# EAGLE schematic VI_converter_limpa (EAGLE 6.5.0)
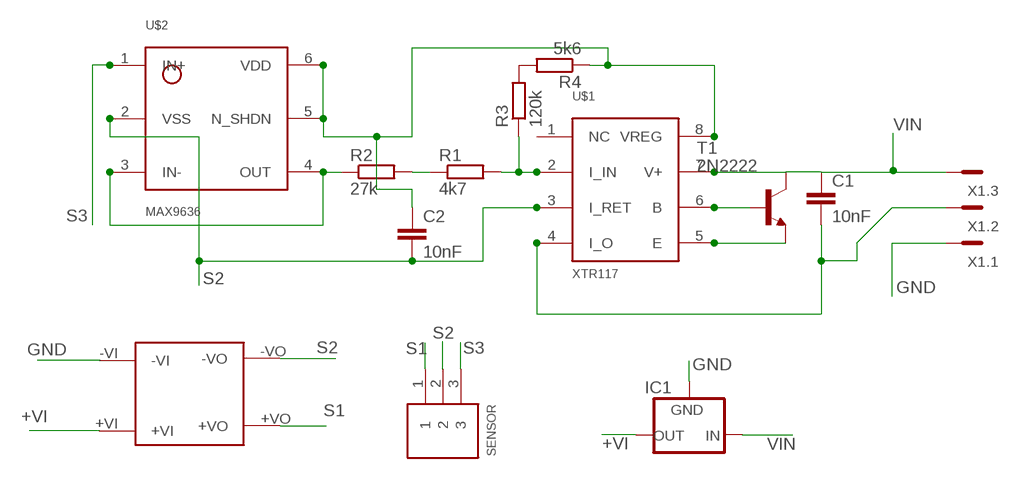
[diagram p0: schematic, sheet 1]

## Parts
C1  10nF  C-EUC1206  [C1206]
C2  10nF  C-EUC1206  [C1206]
IC1  78XXS  [78XXS]
R1  4k7  R-EU_M1206  [M1206]
R2  27k  R-EU_M1206  [M1206]
R3  120k  R-EU_M1206  [M1206]
R4  5k6  R-EU_M1206  [M1206]
SENSOR  3PIN  [B3B-PH-K-S]
T1  2N2222  [TO18]
U$1  XTR117  [MSOP8]
U$2  MAX9636  [SOT363]
U$3  ROE-0505S  [ROE-0505S]
X1  MC3  [MC3]

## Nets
GND: C2.2 U$1.3(I_RET) U$2.2(VSS) X1.1
N$1: T1.2(B) U$1.6(B)
N$2: T1.1(E) U$1.5(E)
N$4: R1.2 R3.1 U$1.2(I_IN)
N$5: R1.1 R2.2
N$6: R3.2 R4.2
N$7: C1.2 U$1.4(I_O) X1.2
N$8: R2.1 U$2.3(IN-) U$2.4(OUT)
N$14: C1.1 T1.3(C) U$1.7(V+) X1.3
S3: U$2.1(IN+)
VDD: C2.1 R4.1 U$1.8(VREG) U$2.5(N_SHDN) U$2.6(VDD)
VIN: IC1.IN
Unconnected: IC1.GND IC1.OUT SENSOR.1 SENSOR.2 SENSOR.3 U$1.1(NC) U$3.+VI U$3.+VO U$3.-VI U$3.-VO

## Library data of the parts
C1 C2 = resistor:C-EU: CAPACITOR, European symbol
IC1 = v-reg:78XXS: VOLTAGE REGULATOR
R1-R4 = resistor:R-EU_: RESISTOR, European symbol
SENSOR = jst_eph:3PIN
T1 = transistor:2N2222: NPN TRANSISTOR
U$1 = rpascoal:XTR117
U$2 = rpascoal:MAX9636
U$3 = carpintas:ROE-0505S: ROE-0505S from RECOM Power
X1 = con-phoenix-381_l:MC3: Mini-Combicon 3.81mm horizontal 3-polig (ohne Gegenstecker)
